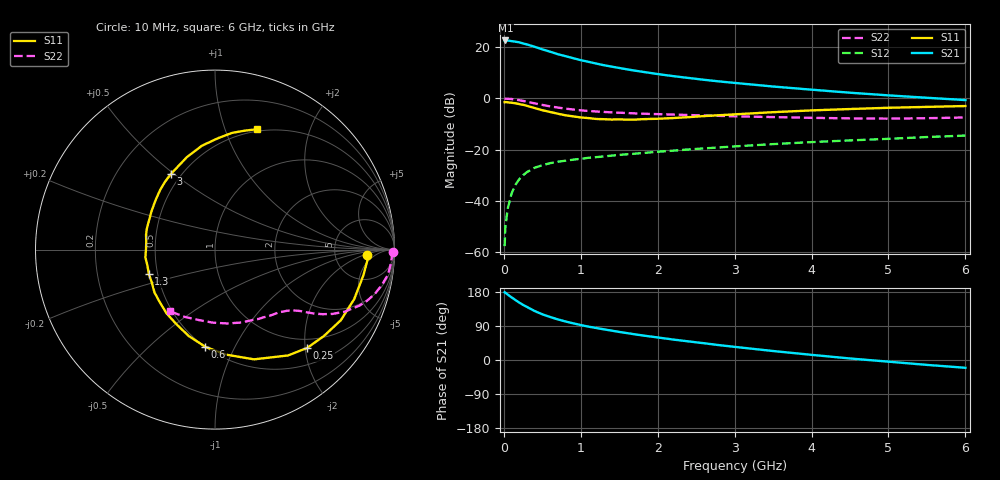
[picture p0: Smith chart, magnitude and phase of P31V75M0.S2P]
! SIEMENS Small Signal Semiconductors
! BFP181
! Si NPN RF Bipolar Junction Transistor in SOT143
! VCE = 1.75 V  IC = 5 mA
! Common Emitter S-Parameters:  March  1996
# GHz  S  MA  R  50
!  f  S11  S21  S12  S22
! GHz  MAG  ANG  MAG  ANG  MAG  ANG  MAG  ANG
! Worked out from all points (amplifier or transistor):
!   36 points, 10 MHz to 6 GHz, reference 50 ohm
!   highest |S21| = 22.6 dB at 20 MHz (marker M1)
!   |S21| within 3 dB of that: start of sweep to 453.3 MHz
!   unconditionally stable (mu >= 1): 1.566 GHz to end of sweep
!   at 250 MHz: K = 0.23, MSG = 25.7 dB, |S12| = -30.0 dB
!   at 1.4 GHz: K = 0.95, MSG = 17.4 dB, |S12| = -22.3 dB
!   at 6 GHz: K = 1.06, MAG = 5.5 dB, |S12| = -14.5 dB
!   S11 on the Smith chart (normalised r, x): 10 MHz: 11, -3; 250 MHz: 0.81, -2.04; 600 MHz: 0.50, -0.77; 1.3 GHz: 0.45, -0.14; 3 GHz: 0.44, +0.49; 6 GHz: 0.48, +1.30
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0.01  0.8458 -2.2  13.53 178.7  0.0013 82.8  0.9895 -0.7
0.02  0.8508 -4.1  13.56 177.5  0.0031 88.7  0.9871 -1.6
0.05  0.8392 -9.8  13.53 172.6  0.007 88.3  0.984 -4.2
0.15  0.804 -29.3  12.84 158.3  0.0205 73.5  0.9503 -12.0
0.2  0.7744 -38.5  12.48 151.6  0.0264 69.7  0.9239 -15.5
0.25  0.7507 -46.9  11.84 145.4  0.0316 65.8  0.894 -18.6
0.3  0.7165 -55.4  11.34 140.1  0.0363 62.1  0.8634 -21.2
0.4  0.649 -70.4  10.21 129.3  0.0442 56.5  0.8006 -25.6
0.5  0.588 -84.1  9.092 120.6  0.0495 51.1  0.7464 -28.7
0.6  0.544 -95.7  8.194 113.6  0.0543 48.1  0.7006 -30.9
0.7  0.5032 -106.9  7.324 107.3  0.0579 45.6  0.6635 -32.6
0.8  0.4686 -117.1  6.703 101.7  0.0607 43.7  0.6322 -33.8
0.9  0.4464 -127.1  6.118 96.9  0.0637 42.0  0.6065 -34.9
1.1  0.413 -144.7  5.188 88.0  0.0693 40.4  0.5691 -36.7
1.3  0.393 -159.8  4.457 80.9  0.0738 39.2  0.5446 -38.6
1.7  0.3854 173.6  3.497 67.9  0.0833 38.2  0.5106 -42.6
2.2  0.4137 148.6  2.727 54.0  0.0954 36.8  0.4834 -48.8
3  0.4884 120.0  2.01 34.7  0.1156 33.4  0.447 -60.9
3.5  0.5387 106.9  1.708 23.7  0.1281 31.0  0.432 -70.1
4.5  0.6207 88.5  1.293 4.0  0.1514 24.7  0.4074 -91.5
5.5  0.683 76.0  1.03 -12.9  0.1761 19.0  0.411 -114.2
6  0.7105 70.7  0.928 -20.6  0.1881 15.4  0.4245 -125.8
